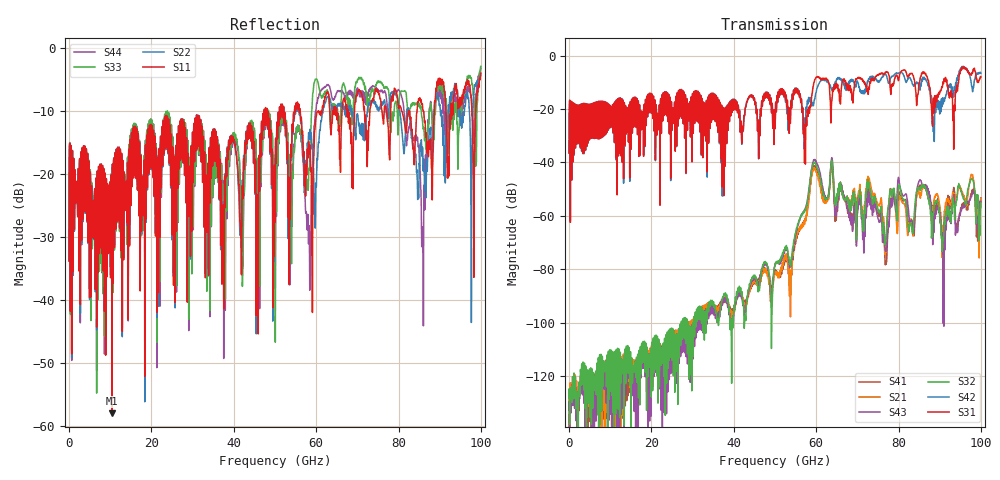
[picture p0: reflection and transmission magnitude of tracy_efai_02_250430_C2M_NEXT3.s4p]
!! PART DESCRIPTION: TE 224G+ VSR Channel- Chip to module, IO connector to CPC(Co-packaged connector) through over the board cable
!! CHANNEL DESCRIPTION: Module trace -> Mated IO 224G+ Connector -> Internal Cable Termination -> 30AWG 300mm Cable -> Cable
!!  termination + CPC connector(No footprint or package included)
!! MODEL REVISION:  Rev 3, Created on April 25, 2025
!! MODEL STATUS: Development
!! MODEL GEOMETRY: 8 Pair Channel
!! MODEL FREQUENCY RANGE: 0 GHz to 100 GHz in 10.00 MHz frequency steps
!! MODEL EDGE RATE LIMITATION: 5ps (Using conservative 0.5/Fmax rule of thumb)
!! PORT DEFINITIONS:
!! Port  1  ----->  Module Side  -->  Host Side, A Row  <-----  Port  2
!! Port  3  ----->  Module Side  -->  Host Side, A Row  <-----  Port  4
# GHz S MA R 45
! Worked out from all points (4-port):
!   10000 points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, 10 MHz to 100 GHz, reference 45 ohm
!   strongest paths, dB at 10 MHz, 25.01 GHz, 50.01 GHz, 75.01 GHz, 100 GHz:
!     S31: -36.5, -27.8, -27.1, -7.4, -8.0
!     S42: -36.5, -28.0, -27.1, -9.9, -6.6
!     S32: -128.3, -113.5, -78.1, -57.9, -56.9
!     S43: -132.7, -118.5, -78.4, -61.0, -54.6
!     S21: -131.4, -110.9, -81.2, -56.0, -53.8
!     S41: -137.1, -113.0, -80.8, -59.1, -53.3
!   lowest |S11| = -58.0 dB at 10.38 GHz (marker M1), VSWR 1.00, Z = 45 + j0.107 ohm
!   |S11| at or under -10 dB: start of sweep to 47.36 GHz; 48.09 GHz to 51.06 GHz (2.963 GHz wide, 5.98 % of centre); 56.14 GHz to 60.39 GHz (4.253 GHz wide, 7.3 % of centre)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
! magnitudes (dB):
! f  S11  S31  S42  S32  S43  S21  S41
! 10 MHz  -33.8  -36.5  -36.5  -128.3  -132.7  -131.4  -137.1
! 10.38 GHz  -58.0  -23.2  -23.2  -123.1  -126.0  -122.7  -121.9
! 53.64 GHz  -22.5  -20.5  -20.2  -76.9  -78.1  -85.3  -85.0
! 59.57 GHz  -13.8  -9.5  -16.5  -40.3  -39.2  -42.6  -41.6
! 76.94 GHz  -9.5  -6.3  -7.2  -68.5  -73.3  -70.8  -78.1
! 85.91 GHz  -9.7  -6.2  -8.2  -48.7  -49.0  -49.1  -49.0
! 100 GHz  -4.0  -8.0  -6.6  -56.9  -54.6  -53.8  -53.3
